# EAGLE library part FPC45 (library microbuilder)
FPC Connector - 45 Pin 0.5mm Bottom Contacts Digikey: 609-1196-1-ND
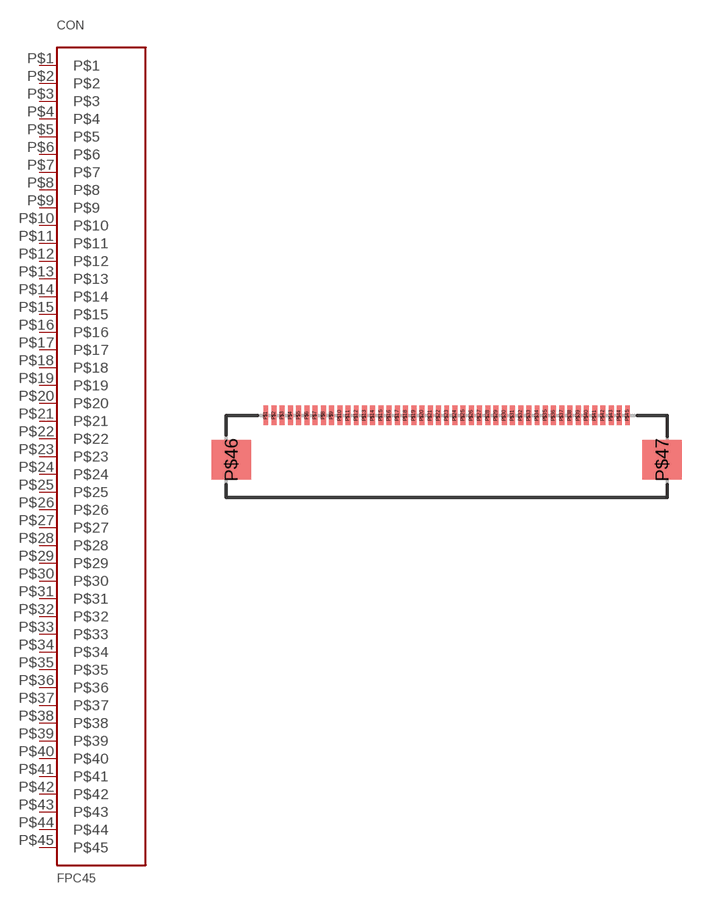
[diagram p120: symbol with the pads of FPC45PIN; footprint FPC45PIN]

Designator prefix CON

## FPC45  [FPC45PIN]
P$1  P$1
P$2  P$2
P$3  P$3
P$4  P$4
P$5  P$5
P$6  P$6
P$7  P$7
P$8  P$8
P$9  P$9
P$10  P$10
P$11  P$11
P$12  P$12
P$13  P$13
P$14  P$14
P$15  P$15
P$16  P$16
P$17  P$17
P$18  P$18
P$19  P$19
P$20  P$20
P$21  P$21
P$22  P$22
P$23  P$23
P$24  P$24
P$25  P$25
P$26  P$26
P$27  P$27
P$28  P$28
P$29  P$29
P$30  P$30
P$31  P$31
P$32  P$32
P$33  P$33
P$34  P$34
P$35  P$35
P$36  P$36
P$37  P$37
P$38  P$38
P$39  P$39
P$40  P$40
P$41  P$41
P$42  P$42
P$43  P$43
P$44  P$44
P$45  P$45

## Footprint FPC45PIN (pad centres in mm)
45-Pin 0.5mm Pitch Bottom Contacts Digikey: 609-1196-1-ND
smd 0.3 x 1.2: P$1 -11,0; P$2 -10.5,0; P$3 -10,0; P$4 -9.5,0; P$5 -9,0; P$6 -8.5,0; P$7 -8,0; P$8 -7.5,0; P$9 -7,0; P$10 -6.5,0; P$11 -6,0; P$12 -5.5,0; P$13 -5,0; P$14 -4.5,0; P$15 -4,0; P$16 -3.5,0; P$17 -3,0; P$18 -2.5,0; P$19 -2,0; P$20 -1.5,0; P$21 -1,0; P$22 -0.5,0; P$23 0,0; P$24 0.5,0; P$25 1,0; P$26 1.5,0; P$27 2,0; P$28 2.5,0; P$29 3,0; P$30 3.5,0; P$31 4,0; P$32 4.5,0; P$33 5,0; P$34 5.5,0; P$35 6,0; P$36 6.5,0; P$37 7,0; P$38 7.5,0; P$39 8,0; P$40 8.5,0; P$41 9,0; P$42 9.5,0; P$43 10,0; P$44 10.5,0; P$45 11,0
smd 2.4 x 2.4: P$46 -13.1,-2.7; P$47 13.1,-2.7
